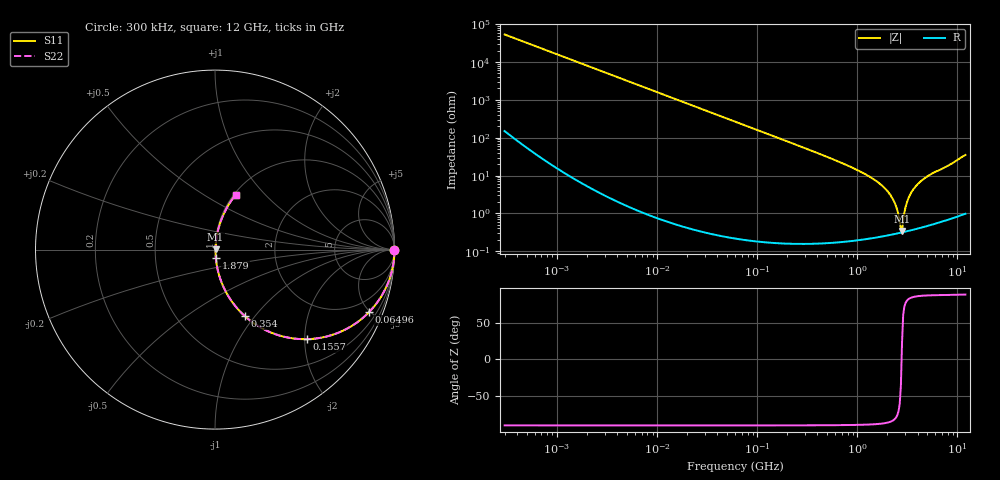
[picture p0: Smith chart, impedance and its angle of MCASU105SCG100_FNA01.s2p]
! MCASU105SCG100_FNA01  S-PARAMETER MODEL  ( Standard Model )
! Model Generated by TAIYO YUDEN Corporation (http://www.ty-top.com)
! Version 1.0
! TAIYO YUDEN Control No. 230609
! Copyright(c) 2023 TAIYO YUDEN CO.,LTD. All Rights Reserved.
! Product Description (link to TY-COMPAS)
! https://ds.yuden.co.jp/TYCOMPAS/or/detail?pn=MCASU105SCG100JFNA01&u=M
! Products Name : Multilayer Ceramic Capacitors
! Characteristics :
!  Capacitance : 10 [pF] , Rated Voltage : 50 [V] , TCC : CG / C0G
!  Case Size : 1.0 x 0.5 / 0.039 x 0.02 [mm/inch] , Thickness : 0.5 / 0.02 [mm/inch]
!  (Conditions: Temperature = 25 [degC] , DC Bias Voltage = 0 [V])
! External Node Assignments :
!  1  o---| |---o  2
! GND o---------o GND
! Frequency Range : 0.3MHz  -  12000MHz  [ 401 STEP ]
# MHZ S RI R 50
! Freq[MHz].  S11 Real  S11 Imag  S21 Real  S21 Imag  S12 Real  S12 Imag  S22 Real  S22 Imag
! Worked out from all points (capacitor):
!   401 points, 300 kHz to 12 GHz, reference 50 ohm
!   read as one part in series: C = 9.9 pF near 316.3 kHz
!   lowest |Z| = 342 mohm at 2.795 GHz (marker M1)
!   series resonance near 2.768 GHz, so ESL is about 330 pH
!   S11 on the Smith chart (normalised r, x): 300 kHz: open; 64.96 MHz: 1.00, -4.94; 155.7 MHz: 1.00, -2.06; 354 MHz: 1.00, -0.89; 1.879 GHz: 1.01, -0.09; 12 GHz: 1.02, +0.70
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0.3  1 -0.00187  8.71e-06 0.00187  8.71e-06 0.00187  1 -0.00187
1.769972  0.9999 -0.011  0.000129 0.011  0.000129 0.011  0.9999 -0.011
10.44266  0.9958 -0.0647  0.00424 0.0647  0.00424 0.0647  0.9958 -0.0647
26.39317  0.9736 -0.1599  0.0264 0.1599  0.0264 0.1599  0.9736 -0.1599
60  0.8773 -0.3276  0.1227 0.3276  0.1227 0.3276  0.8773 -0.3276
64.96309  0.8592 -0.3474  0.1408 0.3474  0.1408 0.3474  0.8592 -0.3474
155.7172  0.5141 -0.499  0.4859 0.499  0.4859 0.499  0.5141 -0.499
353.9943  0.1671 -0.3713  0.8329 0.3713  0.8329 0.3713  0.1671 -0.3713
1048.836  0.0188 -0.1286  0.9812 0.1286  0.9812 0.1286  0.0188 -0.1286
1480.043  0.00822 -0.0769  0.9918 0.0769  0.9918 0.0769  0.00822 -0.0769
1878.541  0.00465 -0.046  0.9954 0.046  0.9954 0.046  0.00465 -0.046
2088.533  0.00377 -0.0332  0.9962 0.0332  0.9962 0.0332  0.00377 -0.0332
2384.334  0.00317 -0.0176  0.9968 0.0176  0.9968 0.0176  0.00317 -0.0176
2514.07  0.00308 -0.0114  0.9969 0.0114  0.9969 0.0114  0.00308 -0.0114
2650.866  0.00307 -0.0053  0.9969 0.0053  0.9969 0.0053  0.00307 -0.0053
2795.104  0.00314 0.00134  0.9969 -0.00134  0.9969 -0.00134  0.00314 0.00134
2870.14  0.00322 0.00561  0.9968 -0.00561  0.9968 -0.00561  0.00322 0.00561
3107.553  0.00368 0.0182  0.9963 -0.0182  0.9963 -0.0182  0.00368 0.0182
3276.641  0.00417 0.0266  0.9958 -0.0266  0.9958 -0.0266  0.00417 0.0266
3944.255  0.00707 0.056  0.9929 -0.056  0.9929 -0.056  0.00707 0.056
5420.343  0.0163 0.106  0.9837 -0.106  0.9837 -0.106  0.0163 0.106
12000  0.1163 0.307  0.8837 -0.307  0.8837 -0.307  0.1163 0.307
